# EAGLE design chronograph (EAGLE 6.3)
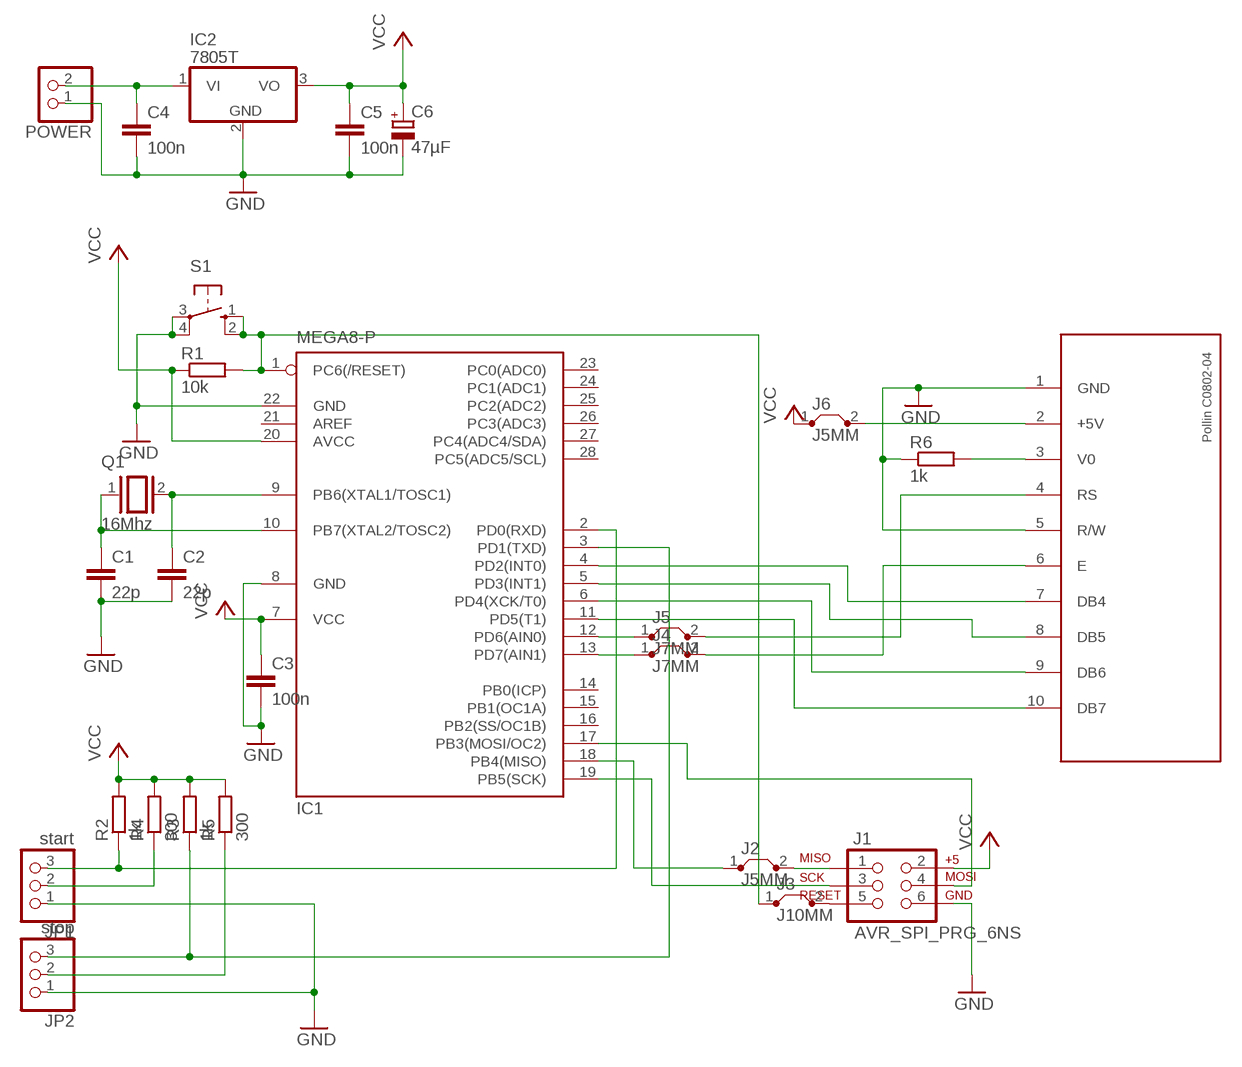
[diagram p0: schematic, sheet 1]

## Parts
C1  22p  C-EU025-024X044  [C025-024X044]
C2  22p  C-EU025-024X044  [C025-024X044]
C3  100n  C-EU050-024X044  [C050-024X044]
C4  100n  C-EU050-024X044  [C050-024X044]
C5  100n  C-EU050-024X044  [C050-024X044]
C6  47µF  CPOL-EUE5-5  [E5-5]
IC1  MEGA8-P  [DIL28-3]
IC2  7805T  [TO220H]
J1  AVR_SPI_PRG_6NS  [2X3-NS]
J2  J5MM  [05]
J3  J10MM  [10]
J4  J7MM  [07]
J5  J7MM  [07]
J6  J5MM  [05]
JP1  start  PINHD-1X3/90  [1X03/90]
JP2  stop  PINHD-1X3/90  [1X03/90]
POWER  PINHD-1X2  [1X02]
Q1  16Mhz  XTAL/S  [QS]
R1  10k  R-EU_0207/12  [0207/12]
R2  1k  R-EU_0207/12  [0207/12]
R3  1k  R-EU_0207/12  [0207/12]
R4  300  R-EU_0207/7  [0207/7]
R5  300  R-EU_0207/7  [0207/7]
R6  1k  R-EU_0207/12  [0207/12]
S1  10-XX  [B3F-10XX]
U$1  POLLIN_LCD  [POLLIN_LCD]

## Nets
GND: C1.2 C2.2 C3.2 C4.2 C5.2 C6.- IC1.8(GND) IC1.22(GND) IC2.2(GND) J1.6 JP1.1 JP2.1 POWER.1 R6.1 S1.3(P) S1.4(P1) U$1.1(GND) U$1.5(R/W)
N$1: J4.2 U$1.6(E)
N$2: IC1.1(PC6(/RESET)) J3.1 R1.2 S1.1(S) S1.2(S1)
N$3: R6.2 U$1.3(V0)
N$4: IC1.4(PD2(INT0)) U$1.7(DB4)
N$5: J5.2 U$1.4(RS)
N$6: IC1.5(PD3(INT1)) U$1.8(DB5)
N$7: C1.1 IC1.10(PB7(XTAL2/TOSC2)) Q1.1
N$8: C2.1 IC1.9(PB6(XTAL1/TOSC1)) Q1.2
N$9: C4.1 IC2.1(VI) POWER.2
N$10: IC1.6(PD4(XCK/T0)) U$1.9(DB6)
N$11: IC1.11(PD5(T1)) U$1.10(DB7)
N$12: J1.1 J2.2
N$13: IC1.18(PB4(MISO)) J2.1
N$14: IC1.19(PB5(SCK)) J1.3
N$15: IC1.17(PB3(MOSI/OC2)) J1.4
N$16: IC1.2(PD0(RXD)) JP1.3 R2.1
N$17: JP1.2 R4.1
N$18: J1.5 J3.2
N$19: IC1.12(PD6(AIN0)) J5.1
N$20: IC1.3(PD1(TXD)) JP2.3 R3.1
N$21: JP2.2 R5.1
N$22: IC1.13(PD7(AIN1)) J4.1
N$23: J6.2 U$1.2(+5V)
VCC: C3.1 C5.1 C6.+ IC1.7(VCC) IC1.20(AVCC) IC2.3(VO) J1.2 J6.1 R1.1 R2.2 R3.2 R4.2 R5.2
Unconnected: IC1.14(PB0(ICP)) IC1.15(PB1(OC1A)) IC1.16(PB2(SS/OC1B)) IC1.21(AREF) IC1.23(PC0(ADC0)) IC1.24(PC1(ADC1)) IC1.25(PC2(ADC2)) IC1.26(PC3(ADC3)) IC1.27(PC4(ADC4/SDA)) IC1.28(PC5(ADC5/SCL))

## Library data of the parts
C1-C5 = rcl:C-EU: CAPACITOR, European symbol
C6 = rcl:CPOL-EU: POLARIZED CAPACITOR, European symbol
IC1 = atmel:MEGA8-P: MICROCONTROLLER 8 Kbytes FLASH, 1 kbytes SRAM, 512 bytes EEPROM, USART, 4-channel 10 bit ADC, 2-channel 8 bit ADC Pin compatible with Atmega48, ATMega88, ATMega168 Source: avr.lbr; OC_FARNELL: unknown; OC_NEWARK: unknown
IC2 = linear:78*: Positive VOLTAGE REGULATOR Source: http://cache.national.com/ds/LM/LM78L05.pdf http://www.fairchildsemi.com/ds/LM/LM7805.pdf
J1 = SparkFun-Connectors:AVR_SPI_PRG_6: AVR ISP 6 Pin This is the reduced ISP connector for AVR programming. Common on Arduino. This footprint will take up less PCB space and can be used with a 10-pin to 6-pin adapter such as SKU: BOB-08508
J2-J6 = jumper:J: Bridge
JP1 JP2 = pinhead:PINHD-1X3: PIN HEADER
POWER = pinhead:PINHD-1X2: PIN HEADER
Q1 = special:XTAL/S: CRYSTAL
R1-R6 = rcl:R-EU_: RESISTOR, European symbol
S1 = switch-omron:10-XX: OMRON SWITCH; MPN: B3F-1000; OC_FARNELL: 176432; OC_NEWARK: 36M3542
U$1 = pollin_lcd:POLLIN_LCD

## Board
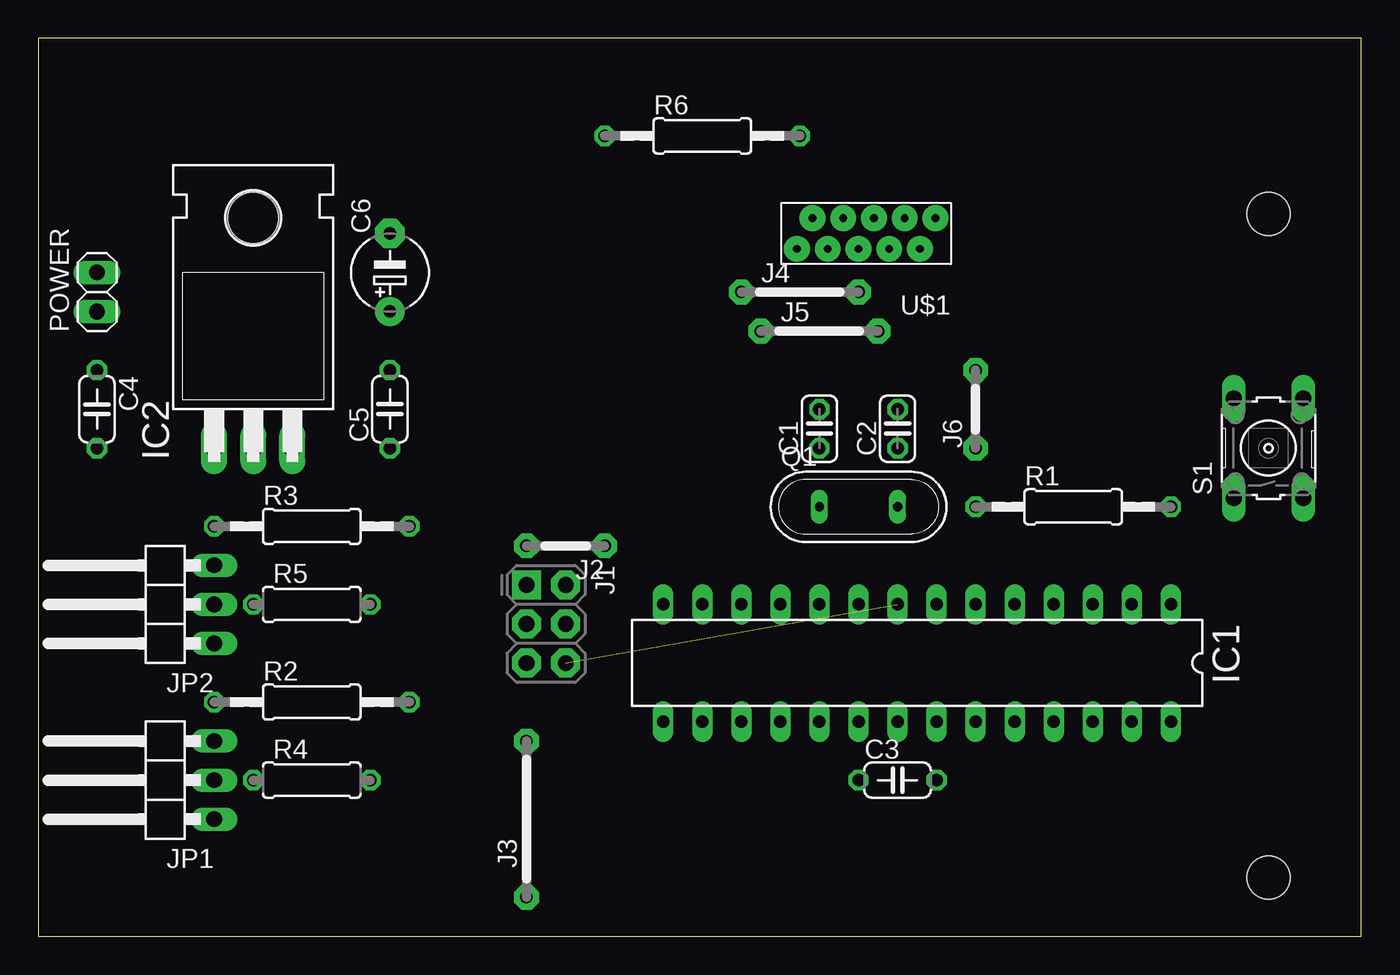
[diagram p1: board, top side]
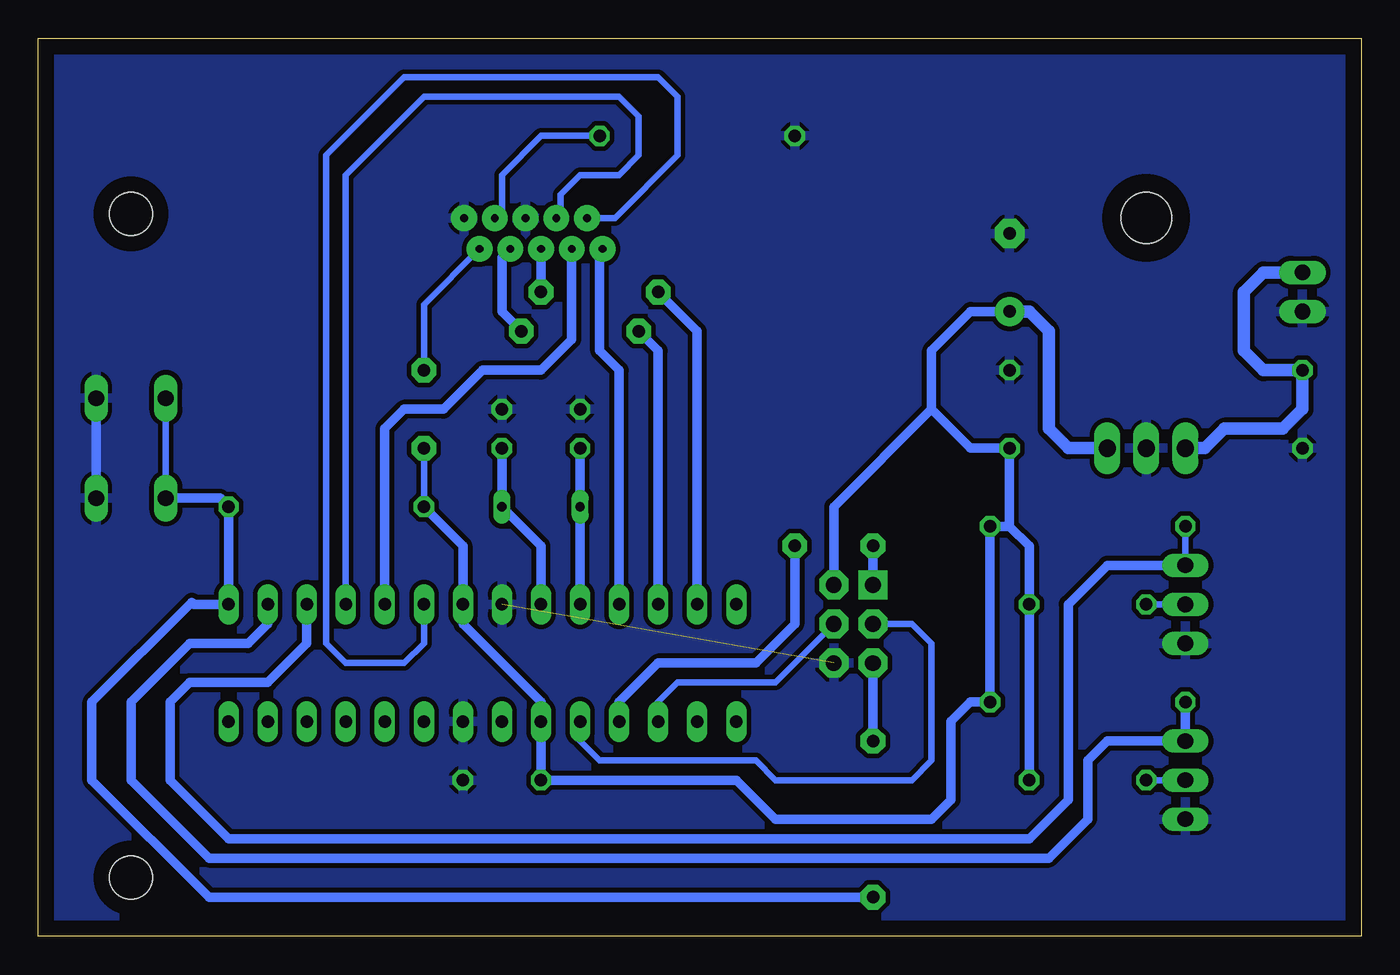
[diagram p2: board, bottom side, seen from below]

Size 86.03 x 58.41 mm. Coordinates in mm from the lower left corner, seen from the top.
Outline: 0,0 86.03,0 86.03,58.41 0,58.41 0,0
Copper layers (1*16): Top 0.035mm / dielectric 1.5mm / Bottom 0.035mm
Design rules "default": minimum track width 10mil, minimum drill 24mil, track to track 8mil, track to pad 8mil, pad to pad 8mil, via to via 8mil, smd to smd 8mil, copper to edge 40mil, drill to drill 8mil, minimum pad ring 10mil, minimum via ring 8mil, stop-mask expansion 4mil, vias tented up to drill 0mil, thermal gap 10mil
Holes 2.8 mm at 80.01,46.99 80.01,3.81

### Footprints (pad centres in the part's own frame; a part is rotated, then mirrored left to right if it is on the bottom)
C025-024X044 = drill 0.813 octagon: 1 -1.27,0; 2 1.27,0
C050-024X044 = drill 0.813 octagon: 1 -2.54,0; 2 2.54,0
E5-5 = drill 0.813 pad 1.905: + -2.54,0 | drill 0.813 pad 1.905 octagon: - 2.54,0
DIL28-3 = drill 0.813 long: 1 -16.51,-3.81; 2 -13.97,-3.81; 3 -11.43,-3.81; 4 -8.89,-3.81; 5 -6.35,-3.81; 6 -3.81,-3.81; 7 -1.27,-3.81; 8 1.27,-3.81; 9 3.81,-3.81; 10 6.35,-3.81; 11 8.89,-3.81; 12 11.43,-3.81; 13 13.97,-3.81; 14 16.51,-3.81; 15 16.51,3.81; 16 13.97,3.81; 17 11.43,3.81; 18 8.89,3.81; 19 6.35,3.81; 20 3.81,3.81; 21 1.27,3.81; 22 -1.27,3.81; 23 -3.81,3.81; 24 -6.35,3.81; 25 -8.89,3.81; 26 -11.43,3.81; 27 -13.97,3.81; 28 -16.51,3.81
TO220H = drill 1.118 long: 1 -2.54,-10.16; 2 0,-10.16; 3 2.54,-10.16 | hole 3.302: 0,4.826
2X3-NS = drill 1.016 pad 1.88 square: 1 -2.54,-1.27 | drill 1.016 pad 1.88 octagon: 2 -2.54,1.27; 3 0,-1.27; 4 0,1.27; 5 2.54,-1.27; 6 2.54,1.27
05 = drill 0.813 pad 1.6 octagon: 1 -2.54,0; 2 2.54,0
10 = drill 0.813 pad 1.6 octagon: 1 -5.08,0; 2 5.08,0
07 = drill 0.813 pad 1.6 octagon: 1 -3.81,0; 2 3.81,0
1X03/90 = drill 1.016 long: 1 -2.54,-3.81; 2 0,-3.81; 3 2.54,-3.81
1X02 = drill 1.016 long: 1 -1.27,0; 2 1.27,0
QS = drill 0.61 long: 1 -2.54,0; 2 2.54,0
0207/12 = drill 0.813 octagon: 1 -6.35,0; 2 6.35,0
0207/7 = drill 0.813 octagon: 1 -3.81,0; 2 3.81,0
B3F-10XX = drill 1.016 long: 1 -3.251,2.261; 2 3.251,2.261; 3 -3.251,-2.261; 4 3.251,-2.261
POLLIN_LCD = drill 0.5 pad 1.676: 1 -5,-1; 2 -4,1; 3 -3,-1; 4 -2,1; 5 -1,-1; 6 0,1; 7 1,-1; 8 2,1; 9 3,-1; 10 4,1

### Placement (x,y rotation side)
C1  50.8,33.02 90 top
C2  55.88,33.02 90 top
C3  55.88,10.16 0 top
C4  3.81,34.29 270 top
C5  22.86,34.29 90 top
C6  22.86,43.18 90 top
IC1  57.15,17.78 180 top
IC2  13.97,41.91 0 top
J1  33.02,20.32 270 top
J2  34.29,25.4 180 top
J3  31.75,7.62 90 top
J4  49.53,41.91 0 top
J5  50.8,39.37 0 top
J6  60.96,34.29 90 top
JP1  7.62,10.16 90 top
JP2  7.62,21.59 90 top
POWER  3.81,41.91 90 top
Q1  53.34,27.94 0 top
R1  67.31,27.94 0 top
R2  17.78,15.24 0 top
R3  17.78,26.67 0 top
R4  17.78,10.16 0 top
R5  17.78,21.59 0 top
R6  43.18,52.07 0 top
S1  80.01,31.75 90 top
U$1  53.34,45.72 180 top

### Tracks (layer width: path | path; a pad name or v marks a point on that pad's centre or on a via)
GND  (1 unrouted)
  Bottom 0.61: S1.4 S1.3
  pour Bottom (isolate 0.305): 0,0 86.36,0 86.36,57.15 0,57.15
N$1
  Bottom 0.61: J4.2 U$1.6
N$2
  Bottom 0.406: 75.92,21.59 76.06,21.73 | S1.1 S1.2
  Bottom 0.61: J3.1 74.93,2.54 82.55,10.16 82.55,15.24 76.06,21.73 | S1.1 74.22,28.5 R1.2 IC1.1 75.92,21.59
N$3
  Bottom 0.406: R6.2 53.34,52.07 55.88,49.53 55.88,47.18 U$1.3
N$4
  Bottom 0.406: IC1.4 66.04,49.53 60.96,54.61 48.26,54.61 46.99,53.34 46.99,50.8 48.26,49.53 50.8,49.53 52.07,48.26 52.07,46.99 U$1.7
N$5
  Bottom 0.61: J5.2 55.88,40.64 55.88,44.18 U$1.4
N$6
  Bottom 0.61: U$1.8 51.34,38.83 53.34,36.83 57.15,36.83 59.69,34.29 62.23,34.29 63.5,33.02 IC1.5
N$7
  Bottom 0.61: C1.1 Q1.1 IC1.10
N$8
  Bottom 0.61: C2.1 Q1.2 53.34,25.4 IC1.9
N$9
  Bottom 0.813: POWER.2 6.35,43.18 7.62,41.91 7.62,38.1 6.35,36.83 C4.1 3.81,34.29 5.08,33.02 8.89,33.02 10.16,31.75 IC2.1
N$10
  Bottom 0.406: U$1.9 48.53,46.72 44.45,50.8 44.45,54.61 45.72,55.88 62.23,55.88 67.31,50.8 67.31,19.05 66.04,17.78 62.23,17.78 60.96,19.05 IC1.6
N$11
  Bottom 0.61: IC1.11 48.26,36.83 49.53,38.1 49.53,44.53 U$1.10
N$12
  Bottom 0.61: J2.2 J1.1
N$13
  Bottom 0.61: J2.1 36.83,20.32 39.37,17.78 45.72,17.78 48.26,15.24 IC1.18
N$14
  Bottom 0.406: J1.3 29.21,20.32 27.94,19.05 27.94,11.43 29.21,10.16 38.1,10.16 39.37,11.43 49.53,11.43 50.8,12.7 IC1.19
N$15
  Bottom 0.406: J1.4 38.1,16.51 44.45,16.51 45.72,15.24 IC1.17
N$16
  Bottom 0.61: R2.1 JP1.3 16.51,12.7 17.78,11.43 17.78,7.62 20.32,5.08 74.93,5.08 80.01,10.16 80.01,15.24 76.2,19.05 72.39,19.05 71.12,20.32 IC1.2
N$17
  Bottom 0.406: JP1.2 R4.1
N$18
  Bottom 0.61: J3.2 J1.5
N$19
  Bottom 0.61: IC1.12 45.72,38.1 J5.1
N$20
  Bottom 0.406: R3.1 JP2.3
  Bottom 0.61: JP2.3 16.51,24.13 19.05,21.59 19.05,8.89 21.59,6.35 73.66,6.35 77.47,10.16 77.47,15.24 76.2,16.51 71.12,16.51 68.58,19.05 IC1.3
N$21
  Bottom 0.406: JP2.2 R5.1
N$22
  Bottom 0.61: J4.1 43.18,39.37 IC1.13
N$23
  Bottom 0.406: J6.2 60.96,41.1 U$1.2
VCC
  Bottom 0.406: J6.1 R1.1
  Bottom 0.61: 27.94,34.29 25.4,31.75 C5.1 22.86,26.67 | 27.94,34.29 27.94,38.1 25.4,40.64 C6.+ | J1.2 34.29,27.94 27.94,34.29 | R1.1 58.42,25.4 IC1.7 58.42,20.32 53.34,15.24 IC1.20 C3.1 40.64,10.16 38.1,7.62 27.94,7.62 26.67,8.89 26.67,13.97 25.4,15.24 R2.2 R3.2 22.86,26.67 | R4.2 R5.2 21.59,25.4 22.86,26.67
  Bottom 0.813: IC2.3 19.05,31.75 20.32,33.02 20.32,39.37 21.59,40.64 C6.+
